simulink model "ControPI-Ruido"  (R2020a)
settings: Solver=ode45  StartTime=0.0  StopTime=30  RelTol=1e-3  EnableMultiTasking=on
libraries: simulink x4

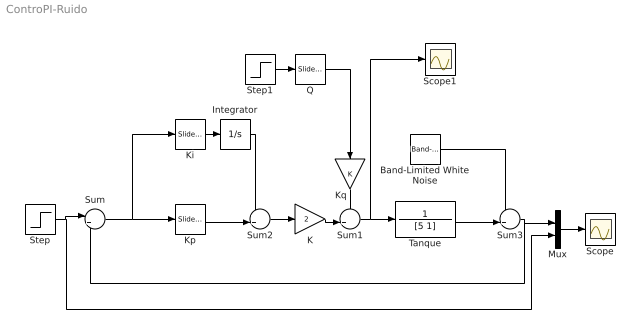
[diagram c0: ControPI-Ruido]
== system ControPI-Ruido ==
  Band-Limited White Noise : simulink/Sources/Band-Limited White Noise  Cov=[1e-5]  Ts=0.1  seed=[23341]
  Integrator : Integrator
  K : Gain  Gain=2
  Ki : simulink/Math Operations/Slider Gain  gain=2.200  low=0  high=20
  Kp : simulink/Math Operations/Slider Gain  gain=4.0  low=0  high=20
  Kq : Gain
  Mux : Mux  Inputs=2
  Q : simulink/Math Operations/Slider Gain  gain=0.450  low=0  high=1
  Scope : Scope
  Scope1 : Scope
  Step : Step  Time=0  SampleTime=0
  Step1 : Step  Time=20
  Sum : Sum  Inputs=|+-
  Sum1 : Sum  Inputs=++|
  Sum2 : Sum  Inputs=++|
  Sum3 : Sum  Inputs=++|
  Tanque : TransferFcn  Numerator=1  Denominator=[5 1]
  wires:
  Sum/1 -> Ki/1, Kp/1
  Mux/1 -> Scope/1
  Step/1 -> Mux/2, Sum/1
  Sum1/1 -> Scope1/1, Tanque/1
  K/1 -> Sum1/2
  Kq/1 -> Sum1/1
  Kp/1 -> Sum2/2
  Integrator/1 -> Sum2/1
  Step1/1 -> Q/1
  Q/1 -> Kq/1
  Sum2/1 -> K/1
  Tanque/1 -> Sum3/2
  Ki/1 -> Integrator/1
  Sum3/1 -> Sum/2, Mux/1
  Band-Limited White Noise/1 -> Sum3/1
